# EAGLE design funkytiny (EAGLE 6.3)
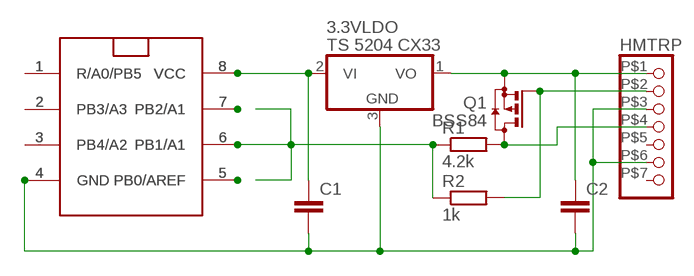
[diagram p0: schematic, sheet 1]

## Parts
3.3VLDO  TS 5204 CX33  78L-SOT23  [SOT23]
ATTINY  ATTINY85  [DIL08]
C1  C-EUC0603  [C0603]
C2  C-EUC0603  [C0603]
HMTRP  PINHD-1X7-RM2  [1X07_RM2]
Q1  BSS84  [SOT23]
R1  4.2k  R-EU_R0603  [R0603]
R2  1k  R-EU_R0603  [R0603]
U$1  ATTINY85SU  [8S2]

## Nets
N$1: HMTRP.P$4 Q1.3(D) R1.2
N$3: 3.3VLDO.1(VO) C2.1 HMTRP.P$1 Q1.2(S)
N$4: HMTRP.P$2 Q1.1(G) R2.2
N$5: 3.3VLDO.3(GND) ATTINY.4(GND) C1.2 C2.2 HMTRP.P$3 HMTRP.P$6 U$1.4(GND)
N$6: 3.3VLDO.2(VI) ATTINY.8(VCC) C1.1 U$1.8(VCC)
N$7: ATTINY.1(R/A0/PB5) U$1.1(R/A0/PB5)
N$8: ATTINY.2(PB3/A3) U$1.2(PB3/A3)
N$9: ATTINY.3(PB4/A2) U$1.3(PB4/A2)
N$10: ATTINY.5(PB0/AREF) U$1.5(PB0/AREF)
N$11: ATTINY.6(PB1/A1) R1.1 R2.1 U$1.6(PB1/A1)
N$12: ATTINY.7(PB2/A1) U$1.7(PB2/A1)
Unconnected: HMTRP.P$5 HMTRP.P$7

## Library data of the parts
3.3VLDO = linear:78L-SOT23
ATTINY = atmel:ATTINY85
C1 C2 = rcl:C-EU: CAPACITOR, European symbol
HMTRP = pinhead:PINHD-1X7-RM2: Pinhead 7x1 RM 2mm
Q1 = transistor-small-signal:BSS84: P-CHANNEL MOS FET
R1 R2 = rcl:R-EU_: RESISTOR, European symbol
U$1 = atmel:ATTINY85SU

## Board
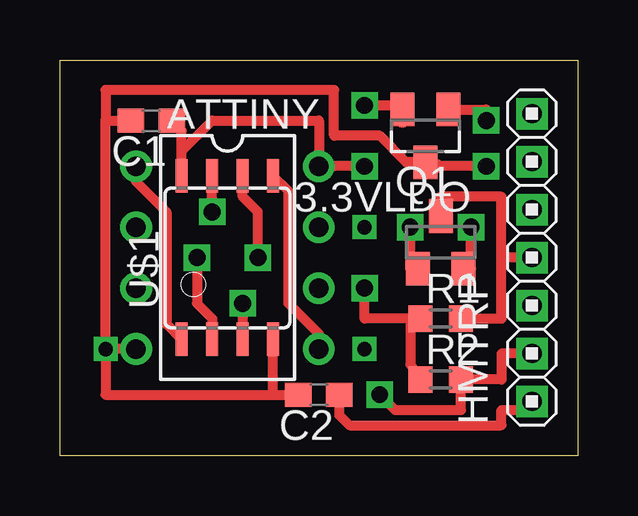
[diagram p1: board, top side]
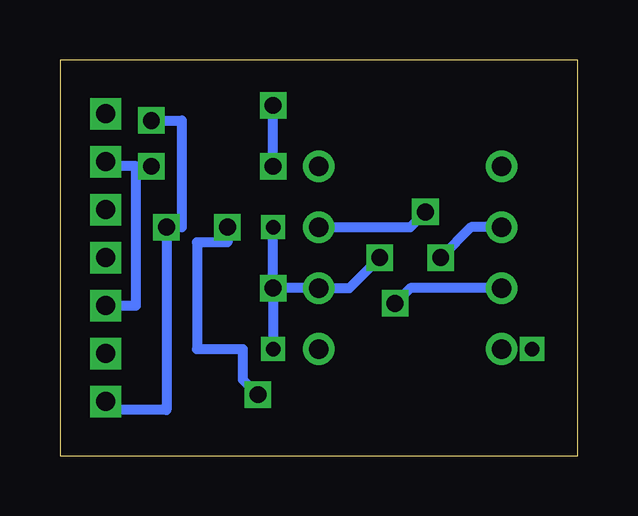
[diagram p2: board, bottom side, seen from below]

Size 21.59 x 16.5 mm. Coordinates in mm from the lower left corner, seen from the top.
Outline: 0,0 0,16.5 21.59,16.5 21.59,0 0,0
Copper layers (1*16): Top 0.035mm / dielectric 1.5mm / Bottom 0.035mm
Design rules "default": minimum track width 10mil, minimum drill 24mil, track to track 8mil, track to pad 8mil, pad to pad 8mil, via to via 8mil, smd to smd 8mil, copper to edge 40mil, drill to drill 8mil, minimum pad ring 10mil, minimum via ring 8mil, stop-mask expansion 4mil, vias tented up to drill 0mil, thermal gap 10mil

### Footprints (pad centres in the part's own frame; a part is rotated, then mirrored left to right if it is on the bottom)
SOT23 = smd 1 x 1.4: 1 -0.95,-1.1; 2 0.95,-1.1; 3 0,1.1
DIL08 = drill 0.813: 1 -3.81,-3.81; 2 -1.27,-3.81; 3 1.27,-3.81; 4 3.81,-3.81; 5 3.81,3.81; 6 1.27,3.81; 7 -1.27,3.81; 8 -3.81,3.81
C0603 = smd 1.1 x 1: 1 -0.85,0; 2 0.85,0
1X07_RM2 = drill 0.8 square: P$1 -6,0; P$2 -4,0; P$3 -2,0; P$4 0,0; P$5 2,0; P$6 4,0; P$7 6,0
R0603 = smd 1 x 1.1: 1 -0.85,0; 2 0.85,0
8S2 = smd 0.5 x 1.4: 1 -1.905,-3.404; 2 -0.645,-3.404; 3 0.625,-3.404; 4 1.895,-3.404; 5 1.905,3.404; 6 0.635,3.404; 7 -0.635,3.404; 8 -1.905,3.404

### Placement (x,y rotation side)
3.3VLDO  15.24,13.34 180 top
ATTINY  6.99,8.26 270 top
C1  3.81,13.97 180 top
C2  10.79,2.54 180 top
HMTRP  19.68,8.26 90 top
Q1  15.88,8.89 0 top
R1  15.88,5.71 0 top
R2  15.88,3.17 0 top
U$1  6.99,8.26 0 top

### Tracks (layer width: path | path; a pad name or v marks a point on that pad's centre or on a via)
N$1
  Top 0.406: HMTRP.P$4 18.41,8.26 | 18.41,8.26 18.41,10.79 15.88,10.79 Q1.3 | R1.2 18.41,5.71 18.41,8.26
N$2  (via drill 0.6)
  other vias: 1.91,4.45
N$3  (via drill 0.7)
  Top 0.406: 3.3VLDO.1 17.78,14.44 v17.78,13.97 | Q1.2 17.14,7.79 v17.14,9.53 | C2.1 11.64,1.69 12.06,1.27 18.41,1.27 18.41,1.91 19.34,1.91 HMTRP.P$1
  Bottom 0.406: v17.78,13.97 16.51,13.97 16.51,9.53 v17.14,9.53 17.14,1.91 19.68,1.91 HMTRP.P$1
N$4  (via drill 0.7)
  Top 0.406: HMTRP.P$2 18.41,4.25 18.41,3.17 R2.2 16.73,1.91 13.97,1.91 v13.34,2.54 | Q1.1 14.61,7.79 v14.61,9.53
  Bottom 0.406: v14.61,9.53 14.61,8.89 15.88,8.89 15.88,4.45 13.97,4.45 13.97,3.17 v13.34,2.54
N$5  (via drill 0.7)
  Top 0.406: 1.91,4.45 1.91,2.54 8.89,2.54 | 8.89,2.54 U$1.4 | 3.3VLDO.3 14.44,12.23 13.34,13.34 11.43,13.34 11.43,15.24 1.91,15.24 1.91,13.97 | ATTINY.4 1.91,4.45 | 1.91,4.45 1.91,13.97 | 8.89,2.54 C2.2 | 1.91,13.97 C1.2 | v17.78,12.06 15.71,12.06
  Top 0.61: 15.71,12.06 3.3VLDO.3
  Bottom 0.406: HMTRP.P$3 18.41,6.25 18.41,12.06 | 18.41,12.06 v17.78,12.06 | 18.41,12.06 19.5,12.06 HMTRP.P$6
N$6  (via drill 0.7)
  Top 0.406: U$1.8 5.08,12.7 | 5.08,12.7 6.35,13.97 10.79,13.97 ATTINY.8 v12.7,12.06 | v12.7,14.61 14.12,14.61 3.3VLDO.2 | 5.08,12.7 5.08,13.55 C1.1
  Top 0.61: 14.29,13.97 3.3VLDO.2
  Bottom 0.406: v12.7,12.06 v12.7,14.61
N$7
  Top 0.406: ATTINY.1 3.17,11.43 4.45,10.16 4.45,5.49 U$1.1
N$8  (via drill 0.7)
  Top 0.406: v5.71,8.26 5.71,6.35 6.35,5.71 U$1.2
  Bottom 0.406: ATTINY.2 4.45,9.53 v5.71,8.26
N$9  (via drill 0.7)
  Top 0.406: v7.62,6.35 U$1.3
  Bottom 0.406: ATTINY.3 6.99,6.99 v7.62,6.35
N$10
  Top 0.406: ATTINY.5 10.79,5.08 9.53,6.35 9.53,11.02 U$1.5
N$11  (via drill 0.6, 0.7)
  Top 0.406: v8.26,8.26 8.26,10.16 7.62,10.79 U$1.6 | R1.1 14.61,5.71 | 14.61,5.71 14.61,3.81 R2.1 | 14.61,5.71 12.7,5.71 v12.7,6.99
  Bottom 0.406: v8.26,8.26 9.53,6.99 ATTINY.6 v12.7,6.99 | v12.7,6.99 v12.7,9.53 | v12.7,6.99 v12.7,4.45
N$12  (via drill 0.7)
  Top 0.406: v6.35,10.16 U$1.7
  Bottom 0.406: ATTINY.7 6.99,9.53 v6.35,10.16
